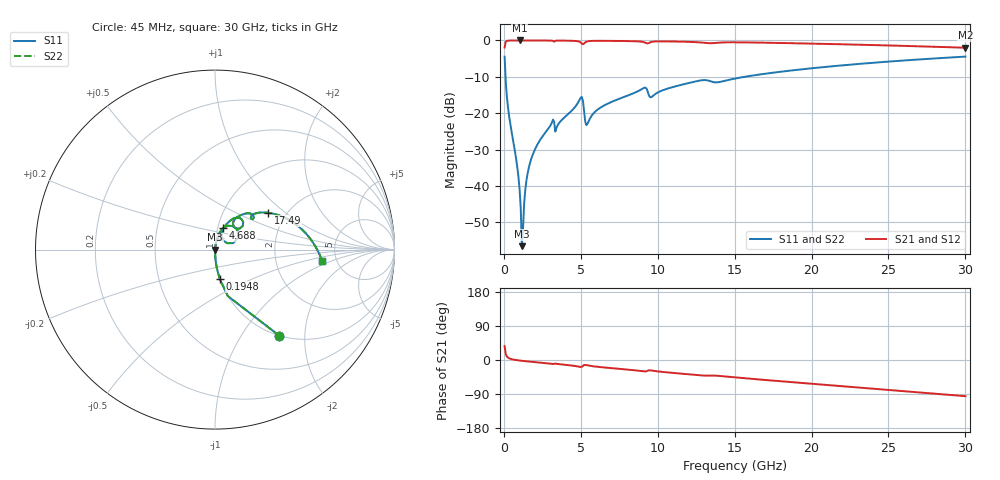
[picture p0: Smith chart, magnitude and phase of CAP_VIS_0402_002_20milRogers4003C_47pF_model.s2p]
! S-parameter model data by Modelithics Inc.  support@modelithics.com  813-866-6335  Tampa FL USA
! S-Parameter data specifications:
! Substrate: 20-mil Rogers 4003C, substrate thickness, H=0.508mm, Dielectric constant, Er=3.75
! PCB Mounting Pad Footprint: Pad width, PadW=0.50mm , Pad length, PadL=0.50mm , Pad gap, PadG (edge-to-edge)=0.40mm , Reference planes=1.4mm apart
! Created Wed Nov 18 12:55:27 2015
# hz S ma R 50
! 2 Port Network Data from SP1.SP block
! freq  magS11  angS11  magS21  angS21  magS12  angS12  magS22  angS22
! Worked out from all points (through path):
!   401 points, 45 MHz to 30 GHz, reference 50 ohm
!   highest |S21| = -0.01 dB at 1.019 GHz (marker M1); lowest = -2.0 dB at 30 GHz (marker M2)
!   group delay of S21, straight-line fit = 8.98 ps
!   lowest |S11| = -56.5 dB at 1.168 GHz (marker M3), VSWR 1.00, Z = 50.1 - j0.116 ohm
!   |S11| at or under -10 dB: 104.6 MHz to 15.64 GHz (15.53 GHz wide, 197 % of centre)
!   |S22| runs from -56.5 to -4.4 dB; largest |S21 - S12| = 0
!   S11 on the Smith chart (normalised r, x): 45 MHz: 1.00, -1.50; 194.8 MHz: 1.00, -0.34; 4.688 GHz: 1.06, +0.26; 17.49 GHz: 1.62, +0.76; 30 GHz: 3.84, -0.74
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4.5e7  0.5992 -53.3  0.8004 36.7  0.8004 36.7  0.5992 -53.3
1.94775e8  0.1662 -80.7  0.9856 9.2  0.9856 9.2  0.1662 -80.7
3.4455e8  0.08937 -85.2  0.9954 4.5  0.9954 4.5  0.08937 -85.2
8.687625e8  0.01825 -87.9  0.9989 -0.6  0.9989 -0.6  0.01825 -87.9
1.018538e9  0.009001 -85.5  0.999 -1.4  0.999 -1.4  0.009001 -85.5
1.168312e9  0.001494 -50.7  0.999 -2.2  0.999 -2.2  0.001494 -50.7
1.318088e9  0.005862 76.9  0.9989 -2.8  0.9989 -2.8  0.005862 76.9
1.617638e9  0.01783 82.2  0.9986 -4.1  0.9986 -4.1  0.01783 82.2
2.066962e9  0.03354 81.9  0.998 -5.8  0.998 -5.8  0.03354 81.9
3.115388e9  0.07396 76.2  0.9924 -10.1  0.9924 -10.1  0.07396 76.2
3.489825e9  0.06829 76.4  0.9939 -10.5  0.9939 -10.5  0.06829 76.4
4.688025e9  0.1269 69.3  0.9817 -16.2  0.9817 -16.2  0.1269 69.3
5.062462e9  0.1675 42.5  0.9067 -18.0  0.9067 -18.0  0.1675 42.5
5.4369e9  0.07198 55.2  0.9723 -14.2  0.9723 -14.2  0.07198 55.2
6.33555e9  0.1216 68.8  0.9876 -19.0  0.9876 -19.0  0.1216 68.8
9.0315e9  0.2188 54.6  0.9538 -29.7  0.9538 -29.7  0.2188 54.6
1.007992e10  0.1965 56.9  0.9711 -30.4  0.9711 -30.4  0.1965 56.9
1.50225e10  0.2994 42.0  0.9429 -45.9  0.9429 -45.9  0.2994 42.0
1.749379e10  0.3606 34.7  0.9265 -54.4  0.9265 -54.4  0.3606 34.7
2.003996e10  0.4152 26.5  0.9041 -62.8  0.9041 -62.8  0.4152 26.5
2.505742e10  0.5131 10.3  0.8524 -79.2  0.8524 -79.2  0.5131 10.3
3e10  0.5994 -5.9  0.7939 -95.4  0.7939 -95.4  0.5994 -5.9
